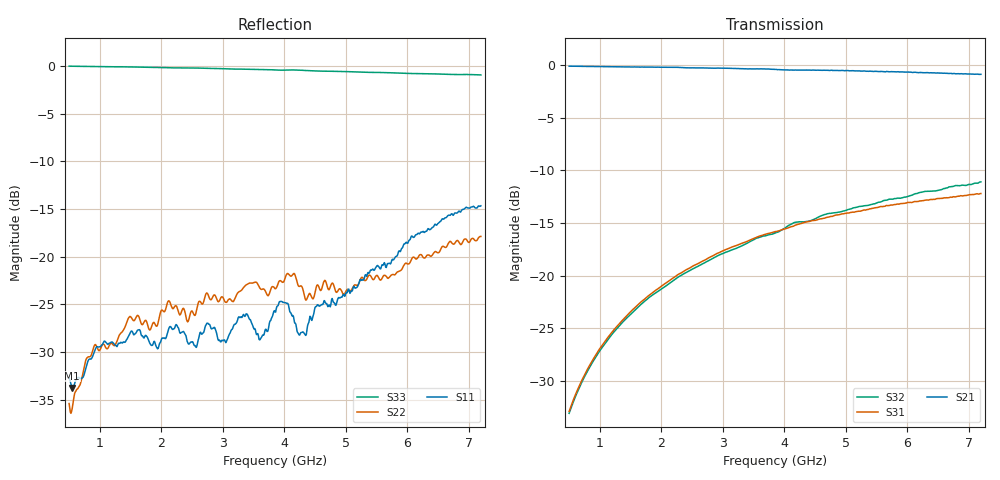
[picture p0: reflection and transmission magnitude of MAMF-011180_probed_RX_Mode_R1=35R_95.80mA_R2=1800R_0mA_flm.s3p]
! MAMF-011180 Probed Data: no bias components
! RX Mode
!  Port 1 =  ANT
!  Port 2 =  RX
!  Port 3 =  TX
! This data represents a typical device, and is provided for engineering reference only.
! This data does not change MACOM's datasheet specifications.
! For questions on this and other MACOM Components, please visit MACOM.com and click on support.
! Technical support requests go to MACOM's application engineering team.
# Hz S  dB  R 50
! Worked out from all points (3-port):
!   671 points, 500 MHz to 7.2 GHz, reference 50 ohm
!   strongest paths, dB at 500 MHz, 2.17 GHz, 3.85 GHz, 5.53 GHz, 7.2 GHz:
!     S21: -0.1, -0.2, -0.4, -0.6, -0.9
!     S31: -32.9, -20.3, -15.8, -13.5, -12.2
!     S32: -33.1, -20.6, -16.0, -13.0, -11.1
!   lowest |S11| = -33.7 dB at 550 MHz (marker M1), VSWR 1.04, Z = 51.7 + j1.27 ohm
!   |S11| at or under -10 dB: start of sweep to end of sweep
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5e8  -32.70 36.9  -0.10 -11.7  -32.93 80.9
     -0.10 -11.7  -35.39 49.9  -33.10 75.6
     -32.92 80.9  -33.10 75.6  -0.03 -12.0
5.5e8  -33.75 36.8  -0.10 -12.8  -32.11 79.8
       -0.10 -12.8  -35.91 36.9  -32.29 74.2
       -32.09 79.8  -32.29 74.3  -0.03 -13.2
9.1e8  -29.97 49.4  -0.13 -21.1  -27.78 73.7
       -0.13 -21.1  -29.32 37.2  -27.97 64.4
       -27.78 73.8  -27.97 64.4  -0.06 -21.8
1.48e9  -28.15 47.3  -0.17 -34.0  -23.57 63.3
        -0.17 -34.0  -26.31 21.3  -23.80 48.6
        -23.56 63.3  -23.80 48.6  -0.10 -35.4
3.37e9  -26.15 43.6  -0.36 -77.4  -16.82 28.5
        -0.35 -77.5  -23.00 -33.8  -17.00 -3.6
        -16.81 28.4  -17.01 -3.6  -0.34 -79.0
3.61e9  -28.66 39.7  -0.37 -82.9  -16.23 24.0
        -0.35 -83.0  -23.34 -43.5  -16.33 -9.0
        -16.23 24.0  -16.35 -9.0  -0.38 -84.2
3.85e9  -25.78 48.9  -0.41 -88.6  -15.83 19.6
        -0.41 -88.6  -23.35 -56.1  -15.97 -16.9
        -15.83 19.5  -15.96 -16.9  -0.42 -89.4
4.34e9  -28.16 68.0  -0.48 -99.7  -14.91 11.0
        -0.48 -99.7  -24.38 -78.7  -14.87 -30.4
        -14.93 11.0  -14.89 -30.4  -0.48 -100.4
5.91e9  -19.14 72.7  -0.67 -137.1  -13.15 -15.6
        -0.65 -137.1  -21.35 -147.7  -12.58 -74.1
        -13.17 -15.5  -12.61 -74.0  -0.76 -134.0
7.2e9  -14.66 59.0  -0.95 -168.6  -12.21 -34.2
       -0.88 -168.8  -17.87 158.8  -11.03 -111.0
       -12.21 -34.4  -11.10 -111.0  -0.94 -160.7
